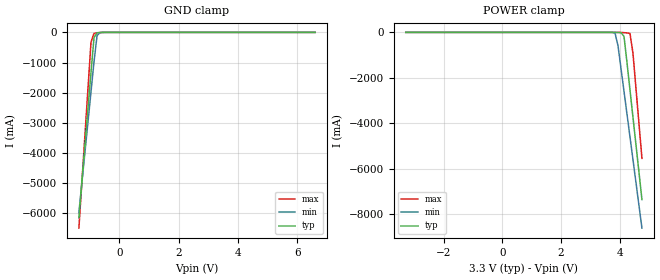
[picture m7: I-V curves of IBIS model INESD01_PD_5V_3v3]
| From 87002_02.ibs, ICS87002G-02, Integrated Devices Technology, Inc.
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[Model] INESD01_PD_5V_3v3
Model_type  Input
Polarity   Non-Inverting
Vinl = 0.8V
Vinh = 2.0V
|   typ   min   max
C_comp   2pF   1.5pF   2.5pF
|   typ   min   max
[Voltage range]  3.3V   3.15V   3.45V
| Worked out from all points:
|   GND clamp passes 1 mA (typ) near -0.55 V on its own axis
[GND_clamp]
|Voltage   I(typ)   I(min)   I(max)
-1.361V   -6.144A    -5.981A    -6.488A
-952.6mV  -1.327A    -1.975A    -329.1mA
-850.5mV  -175.2mA   -975mA     -32.08mA
-748.5mV  -12.63mA   -105.4mA   -18.35mA
-646.4mV  -3.815mA   -5.31mA    -8.297mA
6.6V      128.6uA    131.6uA    121.8uA
[POWER_clamp]
|Voltage   I(typ)   I(min)   I(max)
-3.3V     128.6uA    128.3uA    124.8uA
3.64V     -12.95uA   -197.2uA   -3.249uA
3.844V    -826.8uA   -31.68mA   -47.07uA
3.946V    -3.815mA   -592.1mA   -573.6uA
4.048V    -12.63mA   -1.591A    -3.867mA
4.151V    -175.2mA   -2.592A    -11.82mA
4.253V    -1.327A    -3.593A    -22.84mA
4.355V    -2.53A     -4.595A    -47.66mA
4.457V    -3.735A    -5.597A    -918.8mA
4.763V    -7.349A    -8.606A    -5.538A
